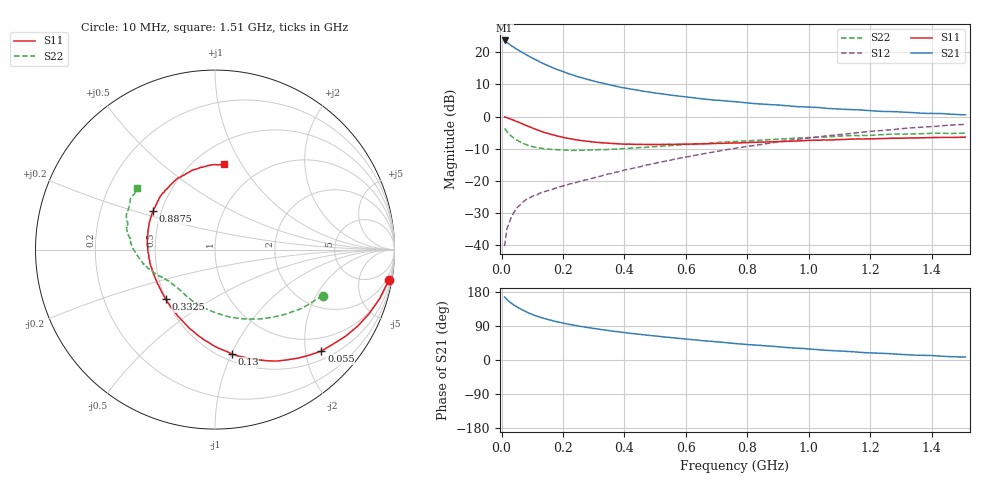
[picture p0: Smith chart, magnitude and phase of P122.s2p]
! Date: Thu Feb 26 08:33:58 1998
# MHZ  S  MA  R  50.0000
!  POLYFET RF DEVICES
!  P122
!  S PARAMETERS
!  VDS=12.5V, IDQ=200mA
! # MHZ S MA R 50
! Freq=MHz Mag[s11] Ang[s11] Mag[s21] Ang[s21] Mag[s12] Ang[s12] Mag[s22] Ang[s22]
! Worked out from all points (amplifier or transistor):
!   201 points, 10 MHz to 1.51 GHz, reference 50 ohm
!   highest |S21| = 23.6 dB at 10 MHz (marker M1)
!   |S21| within 3 dB of that: start of sweep to 54.71 MHz
!   unconditionally stable (mu >= 1): 229.4 MHz to 801.6 MHz; 811.7648 MHz to 813.6494 MHz
!   at 257.5 MHz: K = 1.04, MAG = 14.8 dB, |S12| = -20.0 dB
!   at 760 MHz: K = 1.01, MAG = 6.7 dB, |S12| = -9.9 dB
!   at 1.51 GHz: K = 1.00, MSG = 1.5 dB, |S12| = -2.5 dB
!   S11 on the Smith chart (normalised r, x): 10 MHz: 1, -11; 55 MHz: 0.68, -2.33; 130 MHz: 0.56, -1.00; 332.5 MHz: 0.50, -0.33; 887.5 MHz: 0.45, +0.23; 1.51 GHz: 0.68, +0.84
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10  0.9832 -10.0  15.15 166.1  0.00971 88.1  0.6524 -23.2
17.5  0.9574 -16.6  14.1 159.7  0.01793 73.7  0.5852 -34.0
25  0.9298 -22.6  13.25 154.0  0.0225 70.0  0.5316 -42.7
40  0.873 -33.6  11.84 145.1  0.03229 65.5  0.4628 -56.6
55  0.819 -43.6  10.71 137.7  0.04032 62.7  0.4165 -67.8
77.5  0.7339 -56.8  9.275 128.2  0.05027 60.1  0.3709 -81.9
92.5  0.6879 -64.3  8.46 122.7  0.05488 59.6  0.3503 -90.2
107.5  0.642 -71.6  7.745 117.8  0.05974 58.9  0.3357 -97.3
130  0.5876 -81.0  6.836 111.7  0.06617 59.2  0.3215 -106.5
160  0.5309 -91.7  5.896 104.9  0.07277 60.0  0.3095 -116.0
190  0.4879 -101.2  5.184 99.1  0.081 62.2  0.3036 -122.9
212.5  0.463 -107.6  4.727 95.2  0.08652 63.6  0.3006 -127.2
265  0.42 -120.4  3.942 87.8  0.1008 67.2  0.2982 -135.7
332.5  0.3896 -134.8  3.26 79.6  0.1223 71.0  0.3057 -142.7
392.5  0.3748 -145.6  2.81 73.3  0.1435 72.6  0.3171 -147.3
512.5  0.3672 -164.1  2.274 62.3  0.1941 75.3  0.345 -154.8
655  0.3757 176.5  1.875 50.9  0.2632 75.1  0.3797 -163.4
760  0.3896 163.4  1.695 43.5  0.321 72.7  0.4094 -169.7
887.5  0.4061 148.2  1.52 35.9  0.3947 69.2  0.441 -177.2
1015  0.4272 133.7  1.385 28.2  0.4742 64.2  0.4727 174.6
1262.5  0.4588 106.8  1.193 16.8  0.6189 52.7  0.5292 158.8
1510  0.4772 84.1  1.063 7.7  0.754 40.0  0.5518 141.7
